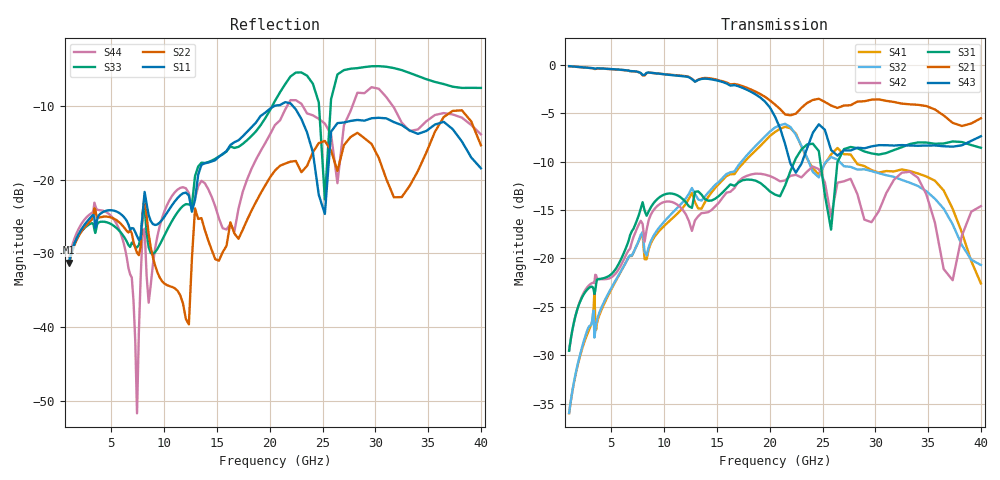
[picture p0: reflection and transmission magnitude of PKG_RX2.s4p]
! Created Mon Sep 18 16:15:26 2017
# hz S ma R 50
! 4 Port Network Data from SP1.SP block
! freq  magS11  angS11  magS12  angS12  magS13  angS13  magS14  angS14
!  magS21  angS21  magS22  angS22  magS23  angS23  magS24  angS24
!  magS31  angS31  magS32  angS32  magS33  angS33  magS34  angS34
!  magS41  angS41  magS42  angS42  magS43  angS43  magS44  angS44
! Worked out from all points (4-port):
!   161 points, 1 GHz to 40 GHz, reference 50 ohm
!   strongest paths, dB at 1 GHz, 2.515 GHz, 6.325 GHz, 15.91 GHz, 40 GHz:
!     S43: -0.1, -0.3, -0.6, -1.9, -7.4
!     S21: -0.1, -0.3, -0.6, -1.8, -5.5
!     S31: -29.5, -23.5, -19.1, -12.8, -8.6
!     S42: -29.5, -23.3, -19.8, -13.2, -14.6
!     S32: -35.9, -28.1, -20.5, -11.3, -20.7
!     S41: -36.0, -28.4, -20.5, -11.5, -22.6
!   lowest |S11| = -31.3 dB at 1 GHz (marker M1), VSWR 1.06, Z = 52.2 + j1.69 ohm
!   |S11| at or under -10 dB: start of sweep to 20.48 GHz; 22.17 GHz to end of sweep
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1e9  0.02734 36.3  0.983 -24.7  0.03342 71.8  0.01588 -119.4
     0.983 -24.7  0.02717 44.8  0.01596 -119.5  0.03349 55.3
     0.03342 71.8  0.01596 -119.5  0.02803 44.5  0.9834 -24.2
     0.01588 -119.4  0.03349 55.3  0.9834 -24.2  0.02986 42.3
7.09732e9  0.04662 -77.9  0.9261 -171.8  0.1425 53.5  0.1073 100.9
           0.9261 -171.8  0.0378 -57.5  0.1075 96.6  0.1291 143.0
           0.1425 53.5  0.1075 96.6  0.03642 -23.3  0.9272 -168.5
           0.1073 100.9  0.1291 143.0  0.9272 -168.5  0.01516 -122.9
1.099864e10  0.07097 -70.3  0.8842 95.0  0.2147 11.3  0.1653 7.1
             0.8842 95.0  0.01838 -54.3  0.1767 -0.8  0.1932 0.2
             0.2147 11.3  0.1767 -0.8  0.05619 -9.0  0.8815 99.6
             0.1653 7.1  0.1932 0.2  0.8815 99.6  0.08185 -48.4
1.484248e10  0.1354 -88.9  0.8413 1.9  0.2035 -5.3  0.2318 -84.3
             0.8413 1.9  0.02889 -50.9  0.2402 -99.2  0.1857 179.8
             0.2035 -5.3  0.2402 -99.2  0.1383 -56.9  0.8335 6.4
             0.2318 -84.3  0.1857 179.8  0.8335 6.4  0.06578 -167.9
2.300123e10  0.2574 114.0  0.5992 -177.1  0.3655 78.2  0.379 26.6
             0.5992 -177.1  0.1122 103.8  0.3823 4.9  0.2621 164.2
             0.3655 78.2  0.3823 4.9  0.5318 89.0  0.3082 -163.1
             0.379 26.6  0.2621 164.2  0.3082 -163.1  0.3262 -174.4
3.033231e10  0.2622 -18.4  0.6628 6.4  0.3439 -8.2  0.2776 -146.2
             0.6628 6.4  0.14 -175.4  0.2756 -173.3  0.1754 176.8
             0.3439 -8.2  0.2756 -173.3  0.5864 -8.1  0.3846 42.4
             0.2776 -146.2  0.1754 176.8  0.3846 42.4  0.4123 -138.2
4e10  0.1193 -100.7  0.5294 141.4  0.3727 -66.7  0.07436 -15.5
      0.5294 141.4  0.171 170.2  0.09256 -45.2  0.1863 65.1
      0.3727 -66.7  0.09256 -45.2  0.4177 -69.6  0.4275 -161.5
      0.07436 -15.5  0.1863 65.1  0.4275 -161.5  0.2026 -138.9
